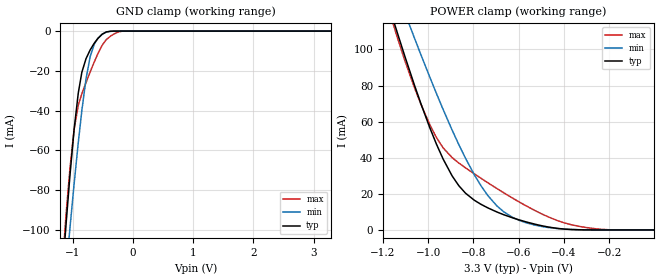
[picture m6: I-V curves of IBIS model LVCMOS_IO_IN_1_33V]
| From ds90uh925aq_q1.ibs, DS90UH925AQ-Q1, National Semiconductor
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[Model] LVCMOS_IO_IN_1_33V
Model_type Input
Vinh = 0.0V
Vinl = 0.0V
C_comp   3.52pF   2.88pF   4.05pF
[Voltage Range]   3.3V   2.97V   3.63V
[Temperature Range]   25.0   130.0   -40.0
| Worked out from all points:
|   GND clamp passes 1 mA (typ) near -0.47 V on its own axis
|   POWER clamp passes 1 mA (typ) near -0.44 V on its own axis
[GND Clamp]
-3.3V     -1.102A    -972.9mA   -1.238A
-1.171V   -123.2mA   -143.1mA   -119.3mA
-1.102V   -95.24mA   -119.1mA   -90.47mA
-1.043V   -72.78mA   -99.22mA   -69.34mA
-973.5mV  -49.48mA   -76.93mA   -49.49mA
-904.2mV  -31.16mA   -56.07mA   -37.28mA
-775.5mV  -13.85mA   -24mA      -25.87mA
-706.2mV  -9.419mA   -12.76mA   -20.5mA
-636.9mV  -6.004mA   -6.452mA   -15.36mA
-438.9mV  -417.3uA   -552.5uA   -4.281mA
-171.6mV  -115.8nA   -1.404uA   -30.72uA
3.293V    1.135nA    0A         -17.45pA
[POWER Clamp]
-3.3V     1.097A     974.8mA    1.228A
-1.162V   119.2mA    140mA      116.8mA
-1.132V   107.4mA    129.9mA    104.8mA
-1.102V   95.8mA     119.9mA    93.42mA
-1.063V   80.87mA    106.9mA    79.44mA
-963.6mV  47.52mA    75.57mA    51.16mA
-894.3mV  29.95mA    55.32mA    40.07mA
-765.6mV  14.13mA    24.25mA    28.52mA
-666.6mV  8.462mA    10.1mA     20.63mA
-567.6mV  4.474mA    3.978mA    13.38mA
-369.6mV  256.4uA    286.7uA    2.963mA
-3.3mV    1.589nA    26.8nA     7.753nA
